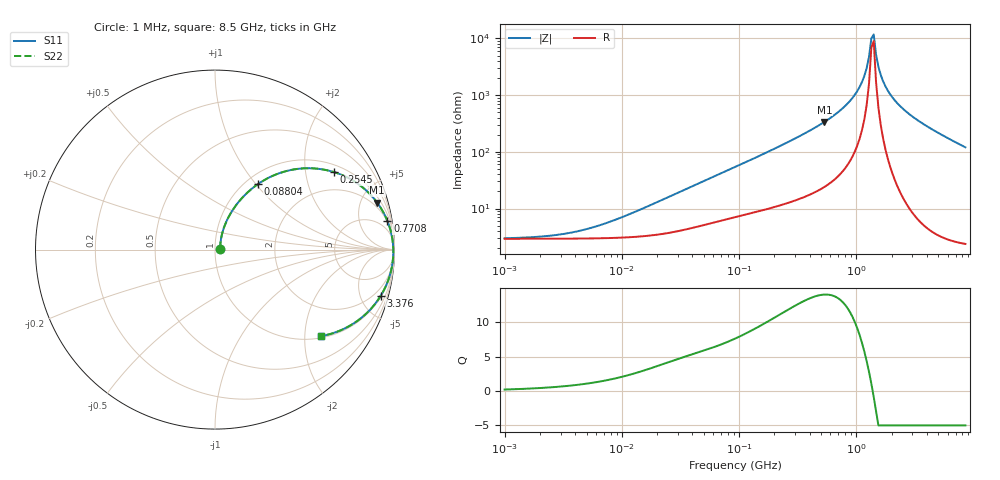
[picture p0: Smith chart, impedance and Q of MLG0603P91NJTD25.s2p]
! S-Parameter Data Generated by TDK Corporation
! Copyright(C) 2025 TDK Corporation.
! All Rights Reserved.
! TDK P/N: MLG0603P91NJTD25 (SMD / SMT Inductor (Coil))
! Property: L=91nH at 300MHz
! Size(LxWxT): 0.6x0.3x0.3mm
! Model Type: s2p (Touchstone File Format Version 1.0)
! Frequency: DC=Yes Start=1MHz Stop=8500MHz 198points Log-sweep
! Model Generated on Feb. 6, 2025
! Terms and conditions regarding TDK Simulation Models:
! 1)This simulation model is being provided solely for informational
!  purposes. Please refer to the specifications of the products in
!  terms of detailed characteristics of such products.
! 2)In no event shall TDK Corporation of any of its subsidiaries be
!  liable for any loss or damage arising, directly or indirectly,
!  from any information contained in this simulation model, including,
!  but not limited to loss or damages arising from any inaccuracies,
!  omissions or errors in connection with such information.
! 3)Any and all copyrights on this simulation model are owned by
!  TDK Corporation.  Duplication or redistribution of this simulation
!  model without prior written permission from TDK Corporation
!  is prohibited.
! 4)This simulation model is subject to any modification or change
!  without any prior notice.
! 5)Neither TDK Corporation nor any of its subsidiaries shall make any
!  warranty, express or implied, including but not limited to the
!  correctness, implied warranties of merchantability and fitness for
!  a particular purpose with respect to this simulation models.
! 6)The use of this simulation model shall be deemed to have consented
!  to the terms and conditions hereof.
! Port Assignments:
!  1 ---@@@--- 2
! Applicable Conditions:
!  Temperature = 25 degC
!  DC Bias Current = 0 A
!  Small Signal Operation
# Hz S MA R 50
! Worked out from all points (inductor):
!   197 points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, 1 MHz to 8.5 GHz, reference 50 ohm
!   read as one part in series: L = 99.4 nH near 15.95 MHz
!   highest Q = 14 at 532.8 MHz (marker M1), where L = 100 nH
!   self-resonance near 1.341 GHz
!   S11 on the Smith chart (normalised r, x): 1 MHz: 1.06, +0.01; 88.04 MHz: 1.14, +1.02; 254.5 MHz: 1.25, +2.89; 770.8 MHz: 2, +12; 3.376 GHz: 1.13, -7.07; 8.5 GHz: 1.05, -2.40
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1000000  0.02904 11.9  0.9716 -0.4  0.9716 -0.4  0.02904 11.9
4587603  0.04019 42.9  0.9709 -1.6  0.9709 -1.6  0.04019 42.9
2.10461e7  0.1302 67.8  0.9585 -7.2  0.9585 -7.2  0.1302 67.8
8.803622e7  0.4345 56.8  0.8447 -25.5  0.8447 -25.5  0.4345 56.8
9.219544e7  0.4494 56.0  0.8366 -26.5  0.8366 -26.5  0.4494 56.0
2.545462e8  0.7921 33.0  0.5466 -52.1  0.5466 -52.1  0.7921 33.0
4.229561e8  0.9071 21.0  0.3596 -64.8  0.3596 -64.8  0.9071 21.0
5.327649e8  0.9404 16.2  0.2797 -69.7  0.2797 -69.7  0.9404 16.2
7.707615e8  0.974 9.4  0.1632 -76.2  0.1632 -76.2  0.974 9.4
9.708683e8  0.9858 5.5  0.0966 -78.8  0.0966 -78.8  0.9858 5.5
1.115076e9  0.9901 3.3  0.05825 -78.6  0.05825 -78.6  0.9901 3.3
1.222927e9  0.992 1.9  0.03322 -75.2  0.03322 -75.2  0.992 1.9
1.280704e9  0.9927 1.1  0.02101 -69.1  0.02101 -69.1  0.9927 1.1
1.34121e9  0.9932 0.4  0.00988 -46.3  0.00988 -46.3  0.9932 0.4
1.404574e9  0.9935 -0.3  0.008444 39.5  0.008444 39.5  0.9935 -0.3
1.470933e9  0.9936 -1.0  0.01908 70.0  0.01908 70.0  0.9936 -1.0
1.540426e9  0.9936 -1.8  0.03129 77.3  0.03129 77.3  0.9936 -1.8
1.689417e9  0.9929 -3.2  0.05656 81.2  0.05656 81.2  0.9929 -3.2
1.940355e9  0.9904 -5.5  0.09562 81.5  0.09562 81.5  0.9904 -5.5
2.444114e9  0.9818 -9.5  0.1643 78.9  0.1643 78.9  0.9818 -9.5
3.37643e9  0.9579 -15.7  0.2708 73.3  0.2708 73.3  0.9579 -15.7
8.5e9  0.7611 -39.3  0.6338 49.5  0.6338 49.5  0.7611 -39.3
